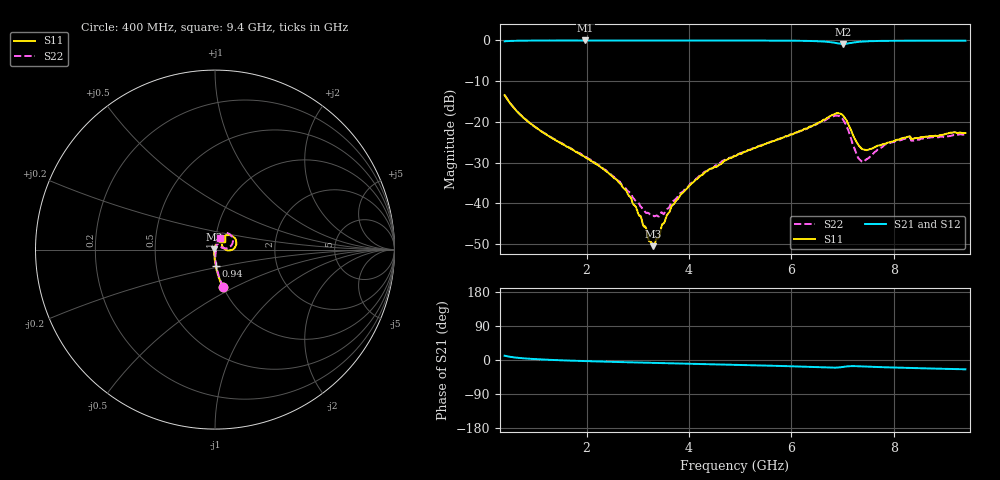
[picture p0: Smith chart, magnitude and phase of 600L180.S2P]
!  American Technical Ceramics  Date:  6/18/2004
!  One Norden Lane
!  Huntington Station,  NY.  11746-2102
!  Tel:  (631) 622-4700  Fax:  (631) 622-4748
!  Part Number  600L180  Mounting Orientation: Vertical
!  Description: Ultra Low ESR Microwave capacitors
!  Application: Coupling, Bypass, Tuning, DC Block
!  Filters, Matching
# GHZ S DB R 50
! Freq  |S11|  S11 Ph  |S21|  S21 Ph  |S12|  S12 Ph  |S22|  S22 Ph
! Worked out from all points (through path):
!   401 points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, 400 MHz to 9.4 GHz, reference 50 ohm
!   highest |S21| = 0.00 dB at 1.975 GHz (marker M1); lowest = -0.9 dB at 7.015 GHz (marker M2)
!   group delay of S21, straight-line fit = 8.77 ps
!   lowest |S11| = -50.6 dB at 3.303 GHz (marker M3), VSWR 1.01, Z = 49.7 + j0.0747 ohm
!   |S11| at or under -10 dB: start of sweep to end of sweep
!   |S22| runs from -43.3 to -13.4 dB; largest |S21 - S12| = 0.0064
!   S11 on the Smith chart (normalised r, x): 400 MHz: 0.99, -0.43; 940 MHz: 0.99, -0.18; 9.4 GHz: 1.08, +0.13
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0.4  -13.45 -78.4  -0.20 11.3  -0.19 11.2  -13.40 -77.8
0.94  -20.78 -87.3  -0.04 2.8  -0.02 2.7  -20.73 -85.4
1.908  -28.23 -94.5  0.00 -2.5  -0.01 -2.6  -28.02 -87.3
1.975  -28.70 -95.6  0.00 -2.9  -0.01 -2.9  -28.55 -86.6
2.448  -32.78 -99.2  -0.01 -4.7  -0.01 -4.7  -32.56 -82.5
2.718  -36.28 -106.1  0.00 -5.6  -0.01 -5.7  -35.86 -75.6
3.123  -45.79 -139.1  0.00 -7.0  -0.01 -7.1  -41.78 -43.1
3.235  -49.45 -160.3  0.00 -7.4  0.00 -7.5  -42.73 -26.1
3.303  -50.56 165.3  -0.01 -7.7  0.00 -7.7  -43.09 -11.7
3.415  -48.38 132.8  -0.01 -8.0  0.00 -8.0  -43.28 6.5
3.685  -40.44 97.1  -0.01 -8.9  -0.01 -8.9  -39.52 43.7
4  -35.81 87.3  -0.01 -9.9  -0.01 -9.9  -35.69 62.7
4.36  -32.11 79.6  -0.02 -11.0  -0.01 -11.1  -32.01 69.1
4.9  -28.40 72.5  -0.02 -12.7  -0.02 -12.7  -28.21 73.0
6.408  -21.06 56.6  -0.14 -18.3  -0.13 -18.0  -21.13 70.5
6.858  -18.02 33.4  -0.60 -20.2  -0.57 -20.2  -18.48 44.8
7.015  -18.54 10.7  -0.85 -18.2  -0.82 -18.2  -19.53 21.2
7.285  -25.22 2.2  -0.38 -16.4  -0.38 -16.4  -28.33 18.1
7.375  -26.60 14.0  -0.28 -16.8  -0.27 -16.8  -29.75 37.4
7.915  -25.03 47.4  -0.09 -19.5  -0.10 -19.5  -25.30 74.1
8.275  -23.68 52.7  -0.07 -20.9  -0.07 -20.8  -24.07 74.2
9.4  -22.75 56.3  -0.06 -24.5  -0.06 -24.4  -22.99 65.2
